(* Logix 5000 AddOnInstructionDefinition export P2M2HBVL_P2HL_AB_BNI00E1_PRM_R0; software revision 31.00 *)

TYPE UDT_P2M2HBVL_P2HL_MSG_Data :
STRUCT
   Read_Parameters : BOOL; {access None}
   Write_AuxVoltageWarnLimits : BOOL; {access None}
   Write_ClearCycleCounts : BOOL; {access None}
   Write_SysCommand : BOOL; {access None}
   AOI_Handshake : BOOL; {access None}
   Write : BOOL; {access None}
   Reset : BOOL; {access None}
   Done : BOOL; {access None}
   Error : BOOL; {access None}
   status : INT; {access None}
   ReceiveData : SINT[97]; {access None}
   SendData : SINT[97]; {access None}
   WriteData : DINT; {access None}
END_STRUCT
END_TYPE

TYPE UDT_P2M2HBVL_P2HL_Parameter_Data :
STRUCT
   Auxiliary_Voltage : INT;
   Error_Channel : DINT;
   Aux_Voltage_High_Warning : INT;
   Aux_Voltage_Low_Warning : INT;
   CycleCount_EV : DINT[25];
   ClearCycleCounts : DINT;
   SystemCommand : INT;
END_STRUCT
END_TYPE

TYPE UDT_P2M2HBVL_P2HL_PRMData :
STRUCT
   P : UDT_P2M2HBVL_P2HL_Parameter_Data;
   M : UDT_P2M2HBVL_P2HL_MSG_Data;
END_STRUCT
END_TYPE

ADD_ON_INSTRUCTION P2M2HBVL_P2HL_AB_BNI00E1_PRM_R0   (* revision 3.0, vendor Parker-Hannifin Corp. *)
// Parker P2M or P2H IO-Link
// Firmware rev >= 1.10
// with Balluff BNI00E1
// IO-Link Master
// Revision note:
// 9/29/2017 Initial release
// 5/14/2018 Limit cycle count, Add system cmd
// 5/24/2018 Separated PD and PRN
// 2/7/2019 Revised to accomodate P2H IOL
VAR_IN_OUT
   Data : UDT_P2M2HBVL_P2HL_PRMData; {required}
   Read_AuxVoltage : MESSAGE; {required}
   Read_AuxVoltLimits : MESSAGE; {required}
   Read_CycleCounts : MESSAGE; {required}
   Read_ErrorChannel : MESSAGE; {required}
   Write_AuxVoltLimits : MESSAGE; {required}
   Write_ClearCounts : MESSAGE; {required}
   Write_SysCommand : MESSAGE; {required}
END_VAR
VAR
   CountTempHolder : DINT; {access None}
   One_Shot : DINT; {access None}
   ReadAuxVoltageComplete : BOOL; {access None}
   ReadAuxVoltLimitsComplete : BOOL; {access None}
   ReadCycleCountsComplete : BOOL; {access None}
   ReadErrorChannelComplete : BOOL; {access None}
   ChTempHolder : DINT; {access None}
END_VAR

ROUTINE Logic   (* ladder *)
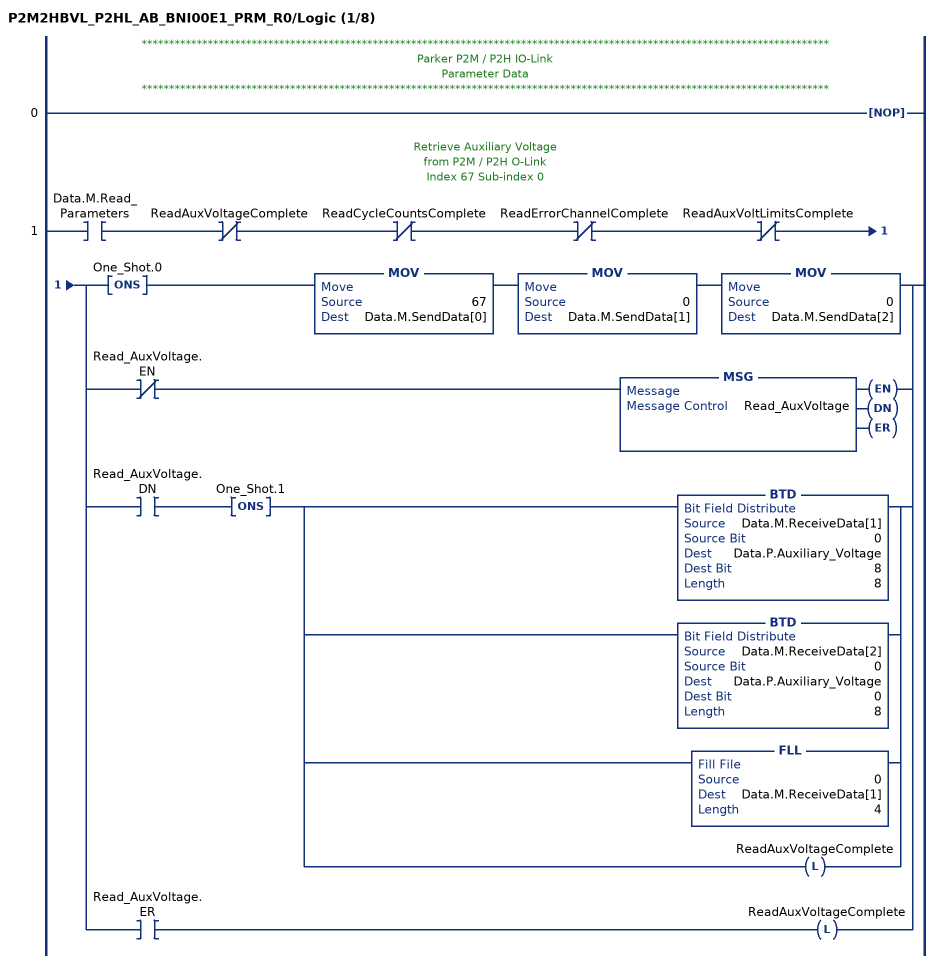
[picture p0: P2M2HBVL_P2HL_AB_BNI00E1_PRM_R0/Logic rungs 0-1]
   // *****************************************************************************************************************************
   // Parker P2M / P2H IO-Link
   // Parameter Data
   // *****************************************************************************************************************************
   0: NOP();
   // Retrieve Auxiliary Voltage
   // from P2M / P2H O-Link
   // Index 67 Sub-index 0
   1: XIC(Data.M.Read_Parameters)XIO(ReadAuxVoltageComplete)XIO(ReadCycleCountsComplete)XIO(ReadErrorChannelComplete)XIO(ReadAuxVoltLimitsComplete)[ONS(One_Shot.0) MOV(67,Data.M.SendData[0]) MOV(0,Data.M.SendData[1]) MOV(0,Data.M.SendData[2]) ,XIO(Read_AuxVoltage.EN) MSG(Read_AuxVoltage) ,XIC(Read_AuxVoltage.DN) ONS(One_Shot.1) [BTD(Data.M.ReceiveData[1],0,Data.P.Auxiliary_Voltage,8,8) ,BTD(Data.M.ReceiveData[2],0,Data.P.Auxiliary_Voltage,0,8) ,FLL(0,Data.M.ReceiveData[1],4) ,OTL(ReadAuxVoltageComplete) ] ,XIC(Read_AuxVoltage.ER) OTL(ReadAuxVoltageComplete) ];
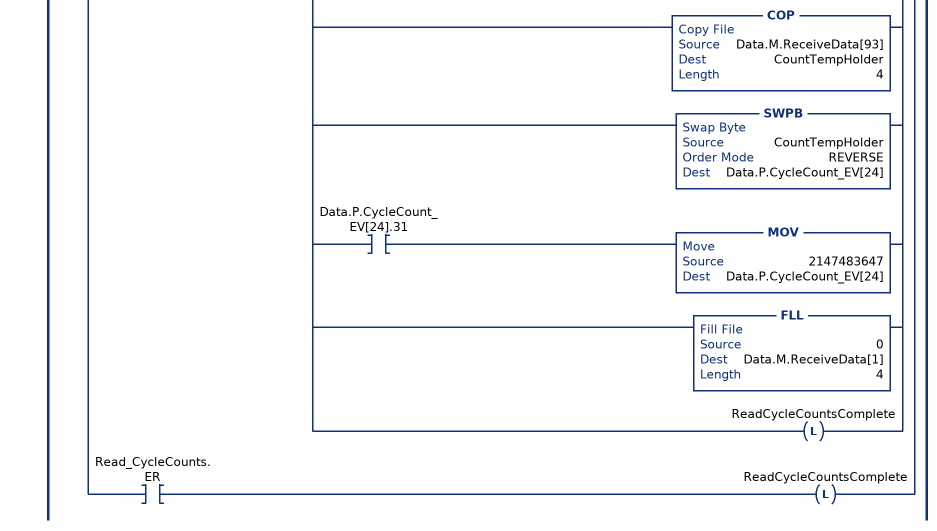
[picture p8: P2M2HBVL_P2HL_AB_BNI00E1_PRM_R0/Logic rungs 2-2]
   // Retrieve Cycle Counts
   // from P2M / P2H IO-Link
   // Index 64 Sub-index 0
   // (Cycle Count is Limited due to Sign Bit)
   2: XIC(Data.M.Read_Parameters)XIC(ReadAuxVoltageComplete)XIO(ReadCycleCountsComplete)XIO(ReadErrorChannelComplete)XIO(ReadAuxVoltLimitsComplete)[ONS(One_Shot.2) MOV(64,Data.M.SendData[0]) MOV(0,Data.M.SendData[1]) MOV(0,Data.M.SendData[2]) ,XIO(Read_CycleCounts.EN) MSG(Read_CycleCounts) ,XIC(Read_CycleCounts.DN) ONS(One_Shot.3) [COP(Data.M.ReceiveData[1],CountTempHolder,4) ,SWPB(CountTempHolder,REVERSE,Data.P.CycleCount_EV[1]) ,XIC(Data.P.CycleCount_EV[1].31) MOV(2147483647,Data.P.CycleCount_EV[1]) ,COP(Data.M.ReceiveData[5],CountTempHolder,4) ,SWPB(CountTempHolder,REVERSE,Data.P.CycleCount_EV[2]) ,XIC(Data.P.CycleCount_EV[2].31) MOV(2147483647,Data.P.CycleCount_EV[2]) ,COP(Data.M.ReceiveData[9],CountTempHolder,4) ,SWPB(CountTempHolder,REVERSE,Data.P.CycleCount_EV[3]) ,XIC(Data.P.CycleCount_EV[3].31) MOV(2147483647,Data.P.CycleCount_EV[3]) ,COP(Data.M.ReceiveData[13],CountTempHolder,4) ,SWPB(CountTempHolder,REVERSE,Data.P.CycleCount_EV[4]) ,XIC(Data.P.CycleCount_EV[4].31) MOV(2147483647,Data.P.CycleCount_EV[4]) ,COP(Data.M.ReceiveData[17],CountTempHolder,4) ,SWPB(CountTempHolder,REVERSE,Data.P.CycleCount_EV[5]) ,XIC(Data.P.CycleCount_EV[5].31) MOV(2147483647,Data.P.CycleCount_EV[5]) ,COP(Data.M.ReceiveData[21],CountTempHolder,4) ,SWPB(CountTempHolder,REVERSE,Data.P.CycleCount_EV[6]) ,XIC(Data.P.CycleCount_EV[6].31) MOV(2147483647,Data.P.CycleCount_EV[6]) ,COP(Data.M.ReceiveData[25],CountTempHolder,4) ,SWPB(CountTempHolder,REVERSE,Data.P.CycleCount_EV[7]) ,XIC(Data.P.CycleCount_EV[7].31) MOV(2147483647,Data.P.CycleCount_EV[7]) ,COP(Data.M.ReceiveData[29],CountTempHolder,4) ,SWPB(CountTempHolder,REVERSE,Data.P.CycleCount_EV[8]) ,XIC(Data.P.CycleCount_EV[8].31) MOV(2147483647,Data.P.CycleCount_EV[8]) ,COP(Data.M.ReceiveData[33],CountTempHolder,4) ,SWPB(CountTempHolder,REVERSE,Data.P.CycleCount_EV[9]) ,XIC(Data.P.CycleCount_EV[9].31) MOV(2147483647,Data.P.CycleCount_EV[9]) ,COP(Data.M.ReceiveData[37],CountTempHolder,4) ,SWPB(CountTempHolder,REVERSE,Data.P.CycleCount_EV[10]) ,XIC(Data.P.CycleCount_EV[10].31) MOV(2147483647,Data.P.CycleCount_EV[10]) ,COP(Data.M.ReceiveData[41],CountTempHolder,4) ,SWPB(CountTempHolder,REVERSE,Data.P.CycleCount_EV[11]) ,XIC(Data.P.CycleCount_EV[11].31) MOV(2147483647,Data.P.CycleCount_EV[11]) ,COP(Data.M.ReceiveData[45],CountTempHolder,4) ,SWPB(CountTempHolder,REVERSE,Data.P.CycleCount_EV[12]) ,XIC(Data.P.CycleCount_EV[12].31) MOV(2147483647,Data.P.CycleCount_EV[12]) ,COP(Data.M.ReceiveData[49],CountTempHolder,4) ,SWPB(CountTempHolder,REVERSE,Data.P.CycleCount_EV[13]) ,XIC(Data.P.CycleCount_EV[13].31) MOV(2147483647,Data.P.CycleCount_EV[13]) ,COP(Data.M.ReceiveData[53],CountTempHolder,4) ,SWPB(CountTempHolder,REVERSE,Data.P.CycleCount_EV[14]) ,XIC(Data.P.CycleCount_EV[14].31) MOV(2147483647,Data.P.CycleCount_EV[14]) ,COP(Data.M.ReceiveData[57],CountTempHolder,4) ,SWPB(CountTempHolder,REVERSE,Data.P.CycleCount_EV[15]) ,XIC(Data.P.CycleCount_EV[15].31) MOV(2147483647,Data.P.CycleCount_EV[15]) ,COP(Data.M.ReceiveData[61],CountTempHolder,4) ,SWPB(CountTempHolder,REVERSE,Data.P.CycleCount_EV[16]) ,XIC(Data.P.CycleCount_EV[16].31) MOV(2147483647,Data.P.CycleCount_EV[16]) ,COP(Data.M.ReceiveData[65],CountTempHolder,4) ,SWPB(CountTempHolder,REVERSE,Data.P.CycleCount_EV[17]) ,XIC(Data.P.CycleCount_EV[17].31) MOV(2147483647,Data.P.CycleCount_EV[17]) ,COP(Data.M.ReceiveData[69],CountTempHolder,4) ,SWPB(CountTempHolder,REVERSE,Data.P.CycleCount_EV[18]) ,XIC(Data.P.CycleCount_EV[18].31) MOV(2147483647,Data.P.CycleCount_EV[18]) ,COP(Data.M.ReceiveData[73],CountTempHolder,4) ,SWPB(CountTempHolder,REVERSE,Data.P.CycleCount_EV[19]) ,XIC(Data.P.CycleCount_EV[19].31) MOV(2147483647,Data.P.CycleCount_EV[19]) ,COP(Data.M.ReceiveData[77],CountTempHolder,4) ,SWPB(CountTempHolder,REVERSE,Data.P.CycleCount_EV[20]) ,XIC(Data.P.CycleCount_EV[20].31) MOV(2147483647,Data.P.CycleCount_EV[20]) ,COP(Data.M.ReceiveData[81],CountTempHolder,4) ,SWPB(CountTempHolder,REVERSE,Data.P.CycleCount_EV[21]) ,XIC(Data.P.CycleCount_EV[21].31) MOV(2147483647,Data.P.CycleCount_EV[21]) ,COP(Data.M.ReceiveData[85],CountTempHolder,4) ,SWPB(CountTempHolder,REVERSE,Data.P.CycleCount_EV[22]) ,XIC(Data.P.CycleCount_EV[22].31) MOV(2147483647,Data.P.CycleCount_EV[22]) ,COP(Data.M.ReceiveData[89],CountTempHolder,4) ,SWPB(CountTempHolder,REVERSE,Data.P.CycleCount_EV[23]) ,XIC(Data.P.CycleCount_EV[23].31) MOV(2147483647,Data.P.CycleCount_EV[23]) ,COP(Data.M.ReceiveData[93],CountTempHolder,4) ,SWPB(CountTempHolder,REVERSE,Data.P.CycleCount_EV[24]) ,XIC(Data.P.CycleCount_EV[24].31) MOV(2147483647,Data.P.CycleCount_EV[24]) ,FLL(0,Data.M.ReceiveData[1],4) ,OTL(ReadCycleCountsComplete) ] ,XIC(Read_CycleCounts.ER) OTL(ReadCycleCountsComplete) ];
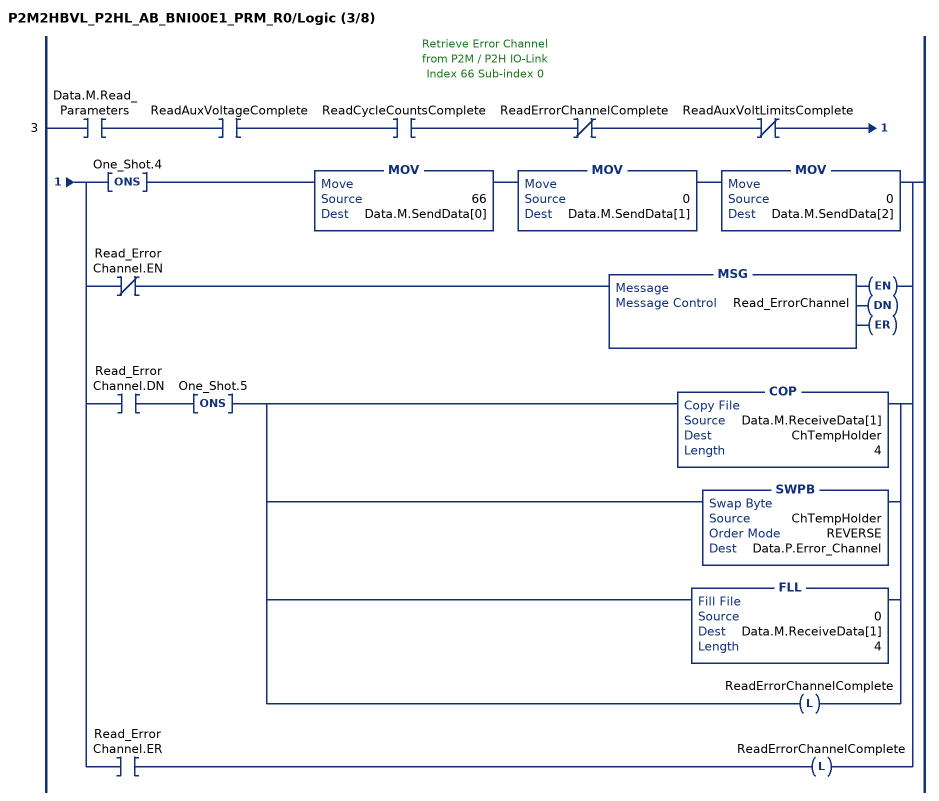
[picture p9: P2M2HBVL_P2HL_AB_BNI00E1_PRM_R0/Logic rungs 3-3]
   // Retrieve Error Channel
   // from P2M / P2H IO-Link
   // Index 66 Sub-index 0
   3: XIC(Data.M.Read_Parameters)XIC(ReadAuxVoltageComplete)XIC(ReadCycleCountsComplete)XIO(ReadErrorChannelComplete)XIO(ReadAuxVoltLimitsComplete)[ONS(One_Shot.4) MOV(66,Data.M.SendData[0]) MOV(0,Data.M.SendData[1]) MOV(0,Data.M.SendData[2]) ,XIO(Read_ErrorChannel.EN) MSG(Read_ErrorChannel) ,XIC(Read_ErrorChannel.DN) ONS(One_Shot.5) [COP(Data.M.ReceiveData[1],ChTempHolder,4) ,SWPB(ChTempHolder,REVERSE,Data.P.Error_Channel) ,FLL(0,Data.M.ReceiveData[1],4) ,OTL(ReadErrorChannelComplete) ] ,XIC(Read_ErrorChannel.ER) OTL(ReadErrorChannelComplete) ];
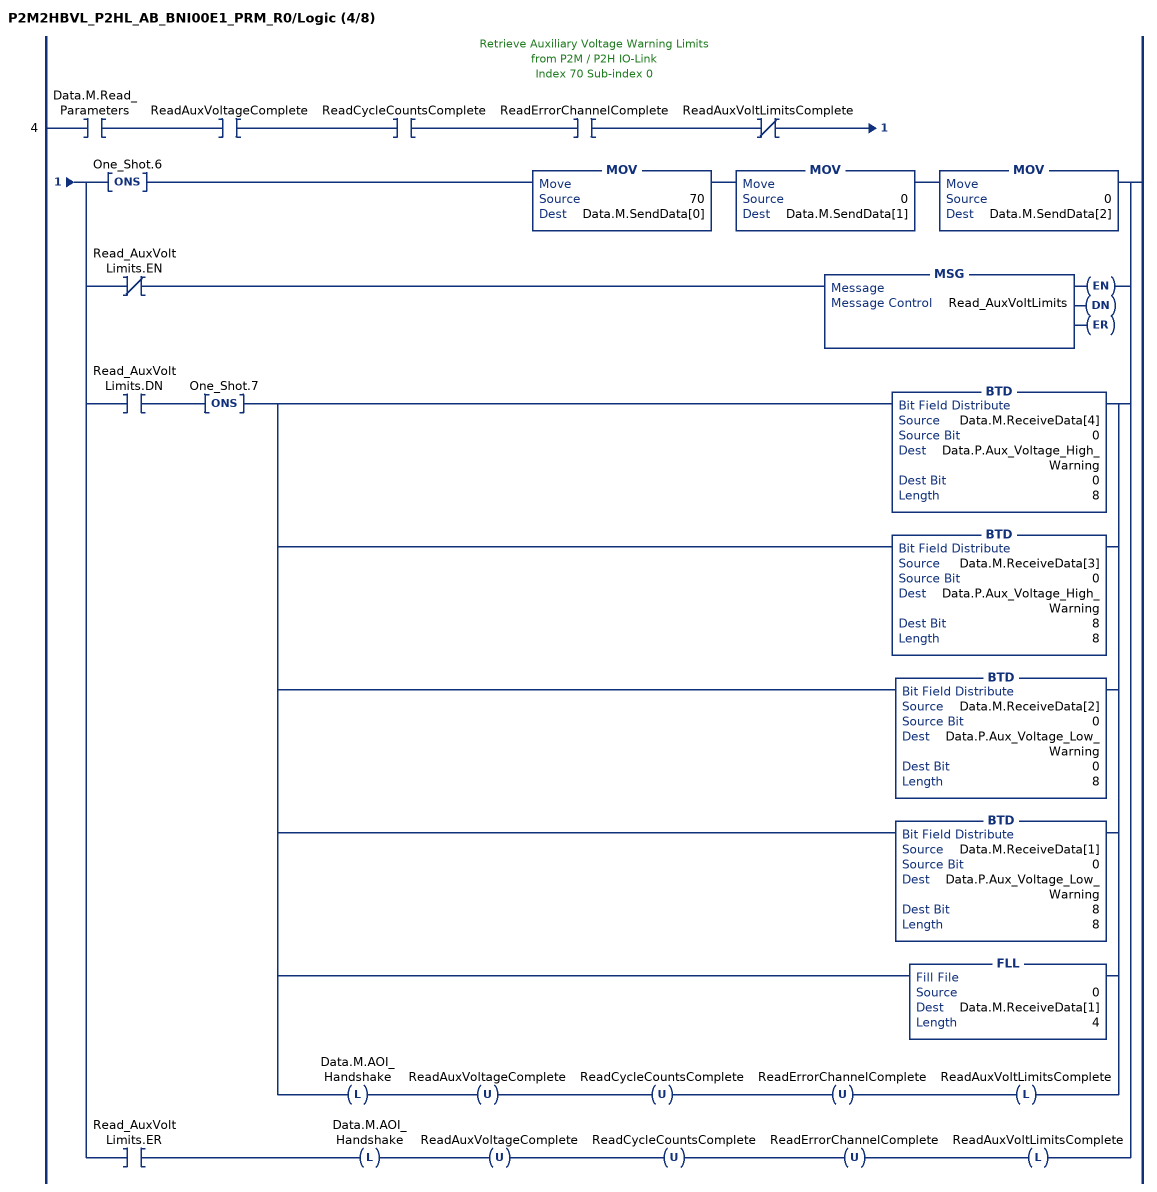
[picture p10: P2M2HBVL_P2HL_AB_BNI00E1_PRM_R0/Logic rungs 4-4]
   // Retrieve Auxiliary Voltage Warning Limits
   // from P2M / P2H IO-Link
   // Index 70 Sub-index 0
   4: XIC(Data.M.Read_Parameters)XIC(ReadAuxVoltageComplete)XIC(ReadCycleCountsComplete)XIC(ReadErrorChannelComplete)XIO(ReadAuxVoltLimitsComplete)[ONS(One_Shot.6) MOV(70,Data.M.SendData[0]) MOV(0,Data.M.SendData[1]) MOV(0,Data.M.SendData[2]) ,XIO(Read_AuxVoltLimits.EN) MSG(Read_AuxVoltLimits) ,XIC(Read_AuxVoltLimits.DN) ONS(One_Shot.7) [BTD(Data.M.ReceiveData[4],0,Data.P.Aux_Voltage_High_Warning,0,8) ,BTD(Data.M.ReceiveData[3],0,Data.P.Aux_Voltage_High_Warning,8,8) ,BTD(Data.M.ReceiveData[2],0,Data.P.Aux_Voltage_Low_Warning,0,8) ,BTD(Data.M.ReceiveData[1],0,Data.P.Aux_Voltage_Low_Warning,8,8) ,FLL(0,Data.M.ReceiveData[1],4) ,OTL(Data.M.AOI_Handshake) OTU(ReadAuxVoltageComplete) OTU(ReadCycleCountsComplete) OTU(ReadErrorChannelComplete) OTL(ReadAuxVoltLimitsComplete) ] ,XIC(Read_AuxVoltLimits.ER) OTL(Data.M.AOI_Handshake) OTU(ReadAuxVoltageComplete) OTU(ReadCycleCountsComplete) OTU(ReadErrorChannelComplete) OTL(ReadAuxVoltLimitsComplete) ];
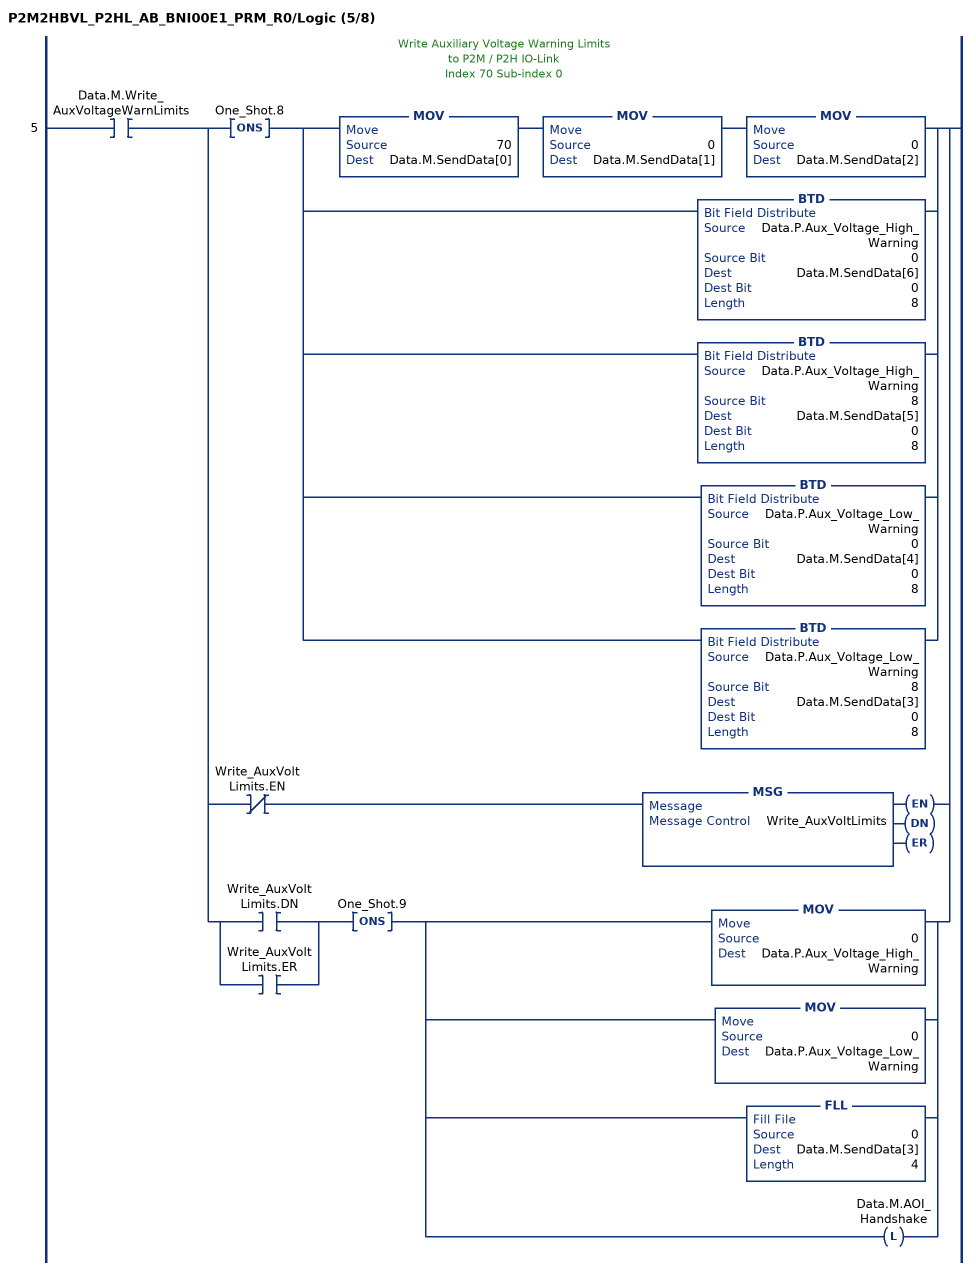
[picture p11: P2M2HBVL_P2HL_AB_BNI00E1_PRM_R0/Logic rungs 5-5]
   // Write Auxiliary Voltage Warning Limits
   // to P2M / P2H IO-Link
   // Index 70 Sub-index 0
   5: XIC(Data.M.Write_AuxVoltageWarnLimits)[ONS(One_Shot.8) [MOV(70,Data.M.SendData[0]) MOV(0,Data.M.SendData[1]) MOV(0,Data.M.SendData[2]) ,BTD(Data.P.Aux_Voltage_High_Warning,0,Data.M.SendData[6],0,8) ,BTD(Data.P.Aux_Voltage_High_Warning,8,Data.M.SendData[5],0,8) ,BTD(Data.P.Aux_Voltage_Low_Warning,0,Data.M.SendData[4],0,8) ,BTD(Data.P.Aux_Voltage_Low_Warning,8,Data.M.SendData[3],0,8) ] ,XIO(Write_AuxVoltLimits.EN) MSG(Write_AuxVoltLimits) ,[XIC(Write_AuxVoltLimits.DN) ,XIC(Write_AuxVoltLimits.ER) ] ONS(One_Shot.9) [MOV(0,Data.P.Aux_Voltage_High_Warning) ,MOV(0,Data.P.Aux_Voltage_Low_Warning) ,FLL(0,Data.M.SendData[3],4) ,OTL(Data.M.AOI_Handshake) ] ];
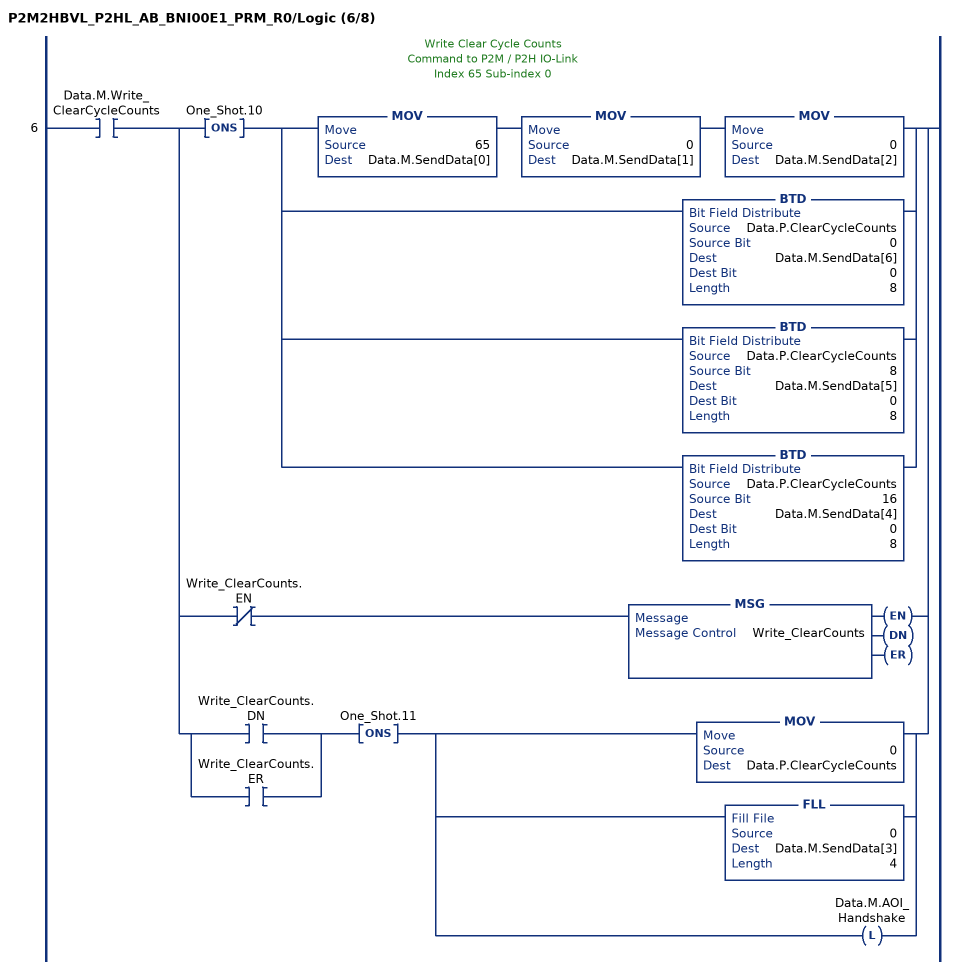
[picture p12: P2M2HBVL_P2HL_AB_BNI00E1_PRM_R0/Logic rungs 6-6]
   // Write Clear Cycle Counts
   // Command to P2M / P2H IO-Link
   // Index 65 Sub-index 0
   6: XIC(Data.M.Write_ClearCycleCounts)[ONS(One_Shot.10) [MOV(65,Data.M.SendData[0]) MOV(0,Data.M.SendData[1]) MOV(0,Data.M.SendData[2]) ,BTD(Data.P.ClearCycleCounts,0,Data.M.SendData[6],0,8) ,BTD(Data.P.ClearCycleCounts,8,Data.M.SendData[5],0,8) ,BTD(Data.P.ClearCycleCounts,16,Data.M.SendData[4],0,8) ] ,XIO(Write_ClearCounts.EN) MSG(Write_ClearCounts) ,[XIC(Write_ClearCounts.DN) ,XIC(Write_ClearCounts.ER) ] ONS(One_Shot.11) [MOV(0,Data.P.ClearCycleCounts) ,FLL(0,Data.M.SendData[3],4) ,OTL(Data.M.AOI_Handshake) ] ];
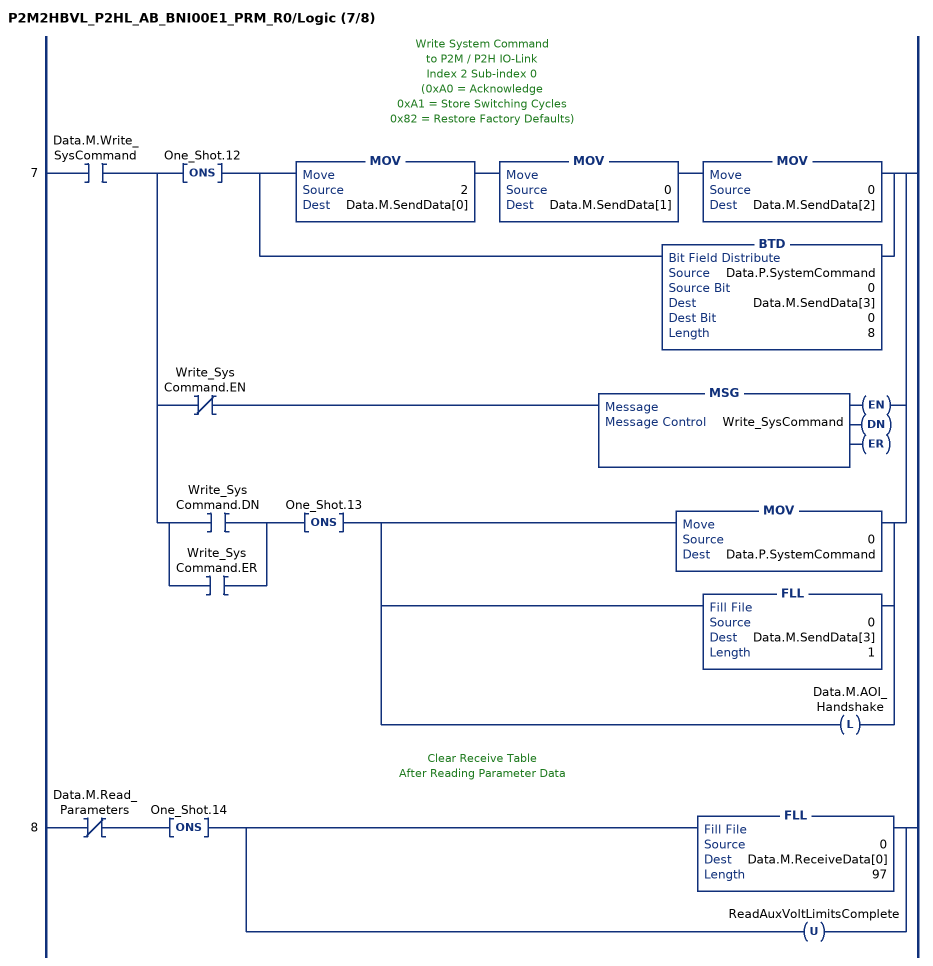
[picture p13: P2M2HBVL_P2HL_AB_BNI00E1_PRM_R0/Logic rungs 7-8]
   // Write System Command
   // to P2M / P2H IO-Link
   // Index 2 Sub-index 0
   // (0xA0 = Acknowledge
   // 0xA1 = Store Switching Cycles
   // 0x82 = Restore Factory Defaults)
   7: XIC(Data.M.Write_SysCommand)[ONS(One_Shot.12) [MOV(2,Data.M.SendData[0]) MOV(0,Data.M.SendData[1]) MOV(0,Data.M.SendData[2]) ,BTD(Data.P.SystemCommand,0,Data.M.SendData[3],0,8) ] ,XIO(Write_SysCommand.EN) MSG(Write_SysCommand) ,[XIC(Write_SysCommand.DN) ,XIC(Write_SysCommand.ER) ] ONS(One_Shot.13) [MOV(0,Data.P.SystemCommand) ,FLL(0,Data.M.SendData[3],1) ,OTL(Data.M.AOI_Handshake) ] ];
   // Clear Receive Table
   // After Reading Parameter Data
   8: XIO(Data.M.Read_Parameters)ONS(One_Shot.14)[FLL(0,Data.M.ReceiveData[0],97) ,OTU(ReadAuxVoltLimitsComplete) ];
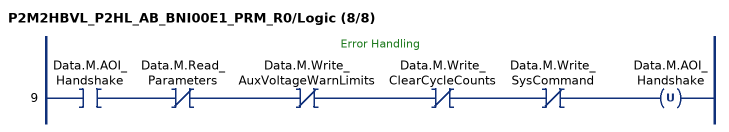
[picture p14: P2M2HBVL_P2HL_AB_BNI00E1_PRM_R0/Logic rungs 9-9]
   // Error Handling
   9: XIC(Data.M.AOI_Handshake)XIO(Data.M.Read_Parameters)XIO(Data.M.Write_AuxVoltageWarnLimits)XIO(Data.M.Write_ClearCycleCounts)XIO(Data.M.Write_SysCommand)OTU(Data.M.AOI_Handshake);
END_ROUTINE
END_ADD_ON_INSTRUCTION
